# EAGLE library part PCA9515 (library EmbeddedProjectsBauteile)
Dual Bidirectional I²C Bus Repeater
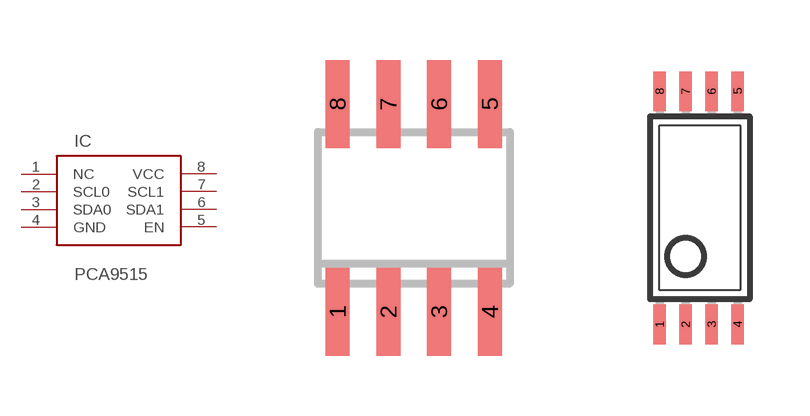
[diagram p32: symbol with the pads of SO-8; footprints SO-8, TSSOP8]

Designator prefix IC

## PCA9515D (EP: 401126)  [SO-8]
1  NC  nc
2  SCL0
3  SDA0
4  GND
5  EN
6  SDA1
7  SCL1
8  VCC  pwr

## PCA9515ADP,APW  [TSSOP8]
Pads as for SO-8

## Footprint SO-8 (pad centres in mm)
smd 0.6 x 2.2: 1 -1.905,-2.6; 2 -0.635,-2.6; 3 0.635,-2.6; 4 1.905,-2.6; 5 1.905,2.6; 6 0.635,2.6; 7 -0.635,2.6; 8 -1.905,2.6

## Footprint TSSOP8 (pad centres in mm)
smd 0.305 x 0.991: 1 -1.005,-2.918; 2 -0.355,-2.918; 3 0.295,-2.918; 4 0.945,-2.918; 5 0.945,2.918; 6 0.295,2.918; 7 -0.355,2.918; 8 -1.005,2.918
